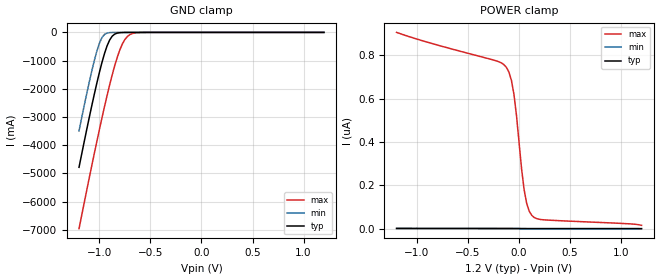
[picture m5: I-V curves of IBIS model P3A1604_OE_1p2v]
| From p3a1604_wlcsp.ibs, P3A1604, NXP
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[Model] P3A1604_OE_1p2v
Model_type Input
Polarity   Non-Inverting
Enable   Active-High
Vinl =  0.526V
Vinh =  0.610V
C_comp   2.027pF   1.667pF   2.300pF
[Model Spec]
Vinh   0.610V   0.505V   0.727V
Vinl   0.526V   0.425V   0.618V
[Temperature Range]   27.000   -40.000   125
[Voltage Range]   1.200V   1.080V   1.320V
[POWER Clamp Reference]   1.200V   1.080V   1.320V
[GND Clamp Reference]   0.0V   0.0V   0.0V
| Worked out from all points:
|   GND clamp passes 1 mA (typ) near -0.70 V on its own axis
[GND_clamp]
|Voltage   I(typ)   I(min)   I(max)
-1.2V     -4.783A    -3.492A    -6.959A
-1.125V   -3.452A    -2.181A    -5.607A
-1.05V    -2.188A    -995.9mA   -4.291A
-1V       -1.414A    -382mA     -3.442A
-975mV    -1.062A    -181.8mA   -3.03A
-925mV    -477.1mA   -23.32mA   -2.237A
-875mV    -134.7mA   -2.896mA   -1.508A
-800mV    -10.35mA   -812.7uA   -619.6mA
-725mV    -1.333mA   -584.8uA   -140.7mA
-675mV    -753.8uA   -466.8uA   -38.67mA
-575mV    -429.3uA   -249.2uA   -2.827mA
1.2V      0A         0A         0A
[POWER_clamp]
|Voltage   I(typ)   I(min)   I(max)
-1.2V     1.361nA    290.9pA    906.2nA
-225mV    983.3pA    150.9pA    775.1nA
-125mV    945.7pA    136.5pA    745.5nA
-75mV     895.5pA    126.8pA    685.4nA
-50mV     830.9pA    117.1pA    620.5nA
-25mV     711.2pA    96.93pA    522.3nA
25mV      365.4pA    30.92pA    275.6nA
50mV      250.4pA    13.81pA    179nA
75mV      191.7pA    7.449pA    116.3nA
100mV     165.3pA    5.299pA    80.38nA
150mV     147.7pA    4.072pA    51.16nA
1.2V      0A         0A         15.41nA
